(* Logix 5000 AddOnInstructionDefinition export AMCI_SV160E2_Disable; software revision 20.03 *)

ADD_ON_INSTRUCTION AMCI_SV160E2_Disable   (* revision 1.0, vendor AMCI *)
// Revision note:
// 8/2019 Version 0 Initial release of SV160E2 Add On Instructions.
// 3/17/20 Version 1 replaced the generic EDS file with a more complete V1.6 EDS file.
VAR_IN_OUT
   AMCI_SV160E2_OUTPUT_DATA : _000A:SV160E2_9125ACD4:O:0; {required}
END_VAR
VAR
   command_data_block : INT[10];
        [0]   // Command Bits MSW
        [1]   // Command Bits LSW
        [2]   // Upper Target Position
        [3]   // Lower Target Position
        [4]   // Upper Programmed Speed
        [5]   // Lower Programmed Speed
END_VAR

ROUTINE Logic   (* ladder *)
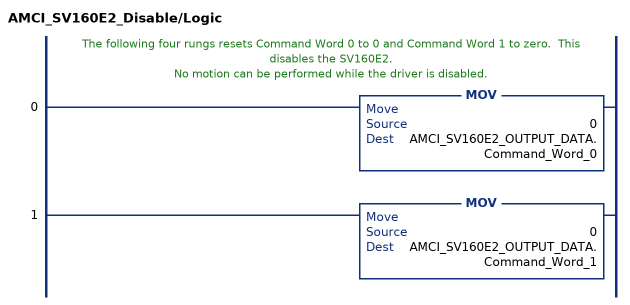
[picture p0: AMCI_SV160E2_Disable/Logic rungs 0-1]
   // The following four rungs resets Command Word 0 to 0 and Command Word 1 to zero.  This disables the SV160E2.
   // No motion can be performed while the driver is disabled.
   0: MOV(0,AMCI_SV160E2_OUTPUT_DATA.Command_Word_0);
   1: MOV(0,AMCI_SV160E2_OUTPUT_DATA.Command_Word_1);
END_ROUTINE
END_ADD_ON_INSTRUCTION
